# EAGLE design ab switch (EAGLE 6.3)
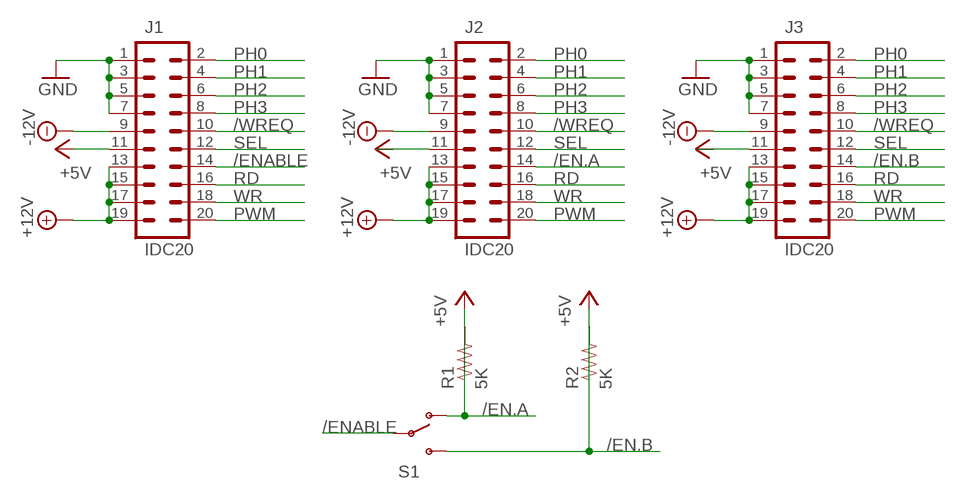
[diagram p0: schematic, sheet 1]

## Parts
J1  IDC20  [IDC20]
J2  IDC20  [IDC20]
J3  IDC20  [IDC20]
R1  5K  RESISTORPTH-1/4W  [AXIAL-0.4]
R2  5K  RESISTORPTH-1/4W  [AXIAL-0.4]
S1  SWITCH-SPDTPTH  [SWITCH-SPDT]

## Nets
+5V: J1.11 J2.11 J3.11 R1.P$1 R2.P$1
+12V: J1.13 J1.15 J1.17 J1.19 J2.13 J2.15 J2.17 J2.19 J3.13 J3.15 J3.17 J3.19
-12V: J1.9 J2.9 J3.9
/EN.A: J2.14 R1.P$2 S1.1(O)
/EN.B: J3.14 R2.P$2 S1.3(S)
/ENABLE: J1.14 S1.2(P)
/WREQ: J1.10 J2.10 J3.10
GND: J1.1 J1.3 J1.5 J1.7 J2.1 J2.3 J2.5 J2.7 J3.1 J3.3 J3.5 J3.7
PH0: J1.2 J2.2 J3.2
PH1: J1.4 J2.4 J3.4
PH2: J1.6 J2.6 J3.6
PH3: J1.8 J2.8 J3.8
PWM: J1.20 J2.20 J3.20
RD: J1.16 J2.16 J3.16
SEL: J1.12 J2.12 J3.12
WR: J1.18 J2.18 J3.18

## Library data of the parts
J1-J3 = big-mess-o-wires:IDC20
R1 R2 = SparkFun-Resistors:RESISTOR: Resistor
S1 = SparkFun-Electromechanical:SWITCH-SPDT: SPDT Switch Simple slide switch, Spark Fun Electronics SKU : COM-00102 DPDT SMT slide switch, AYZ0202, SWCH-08179

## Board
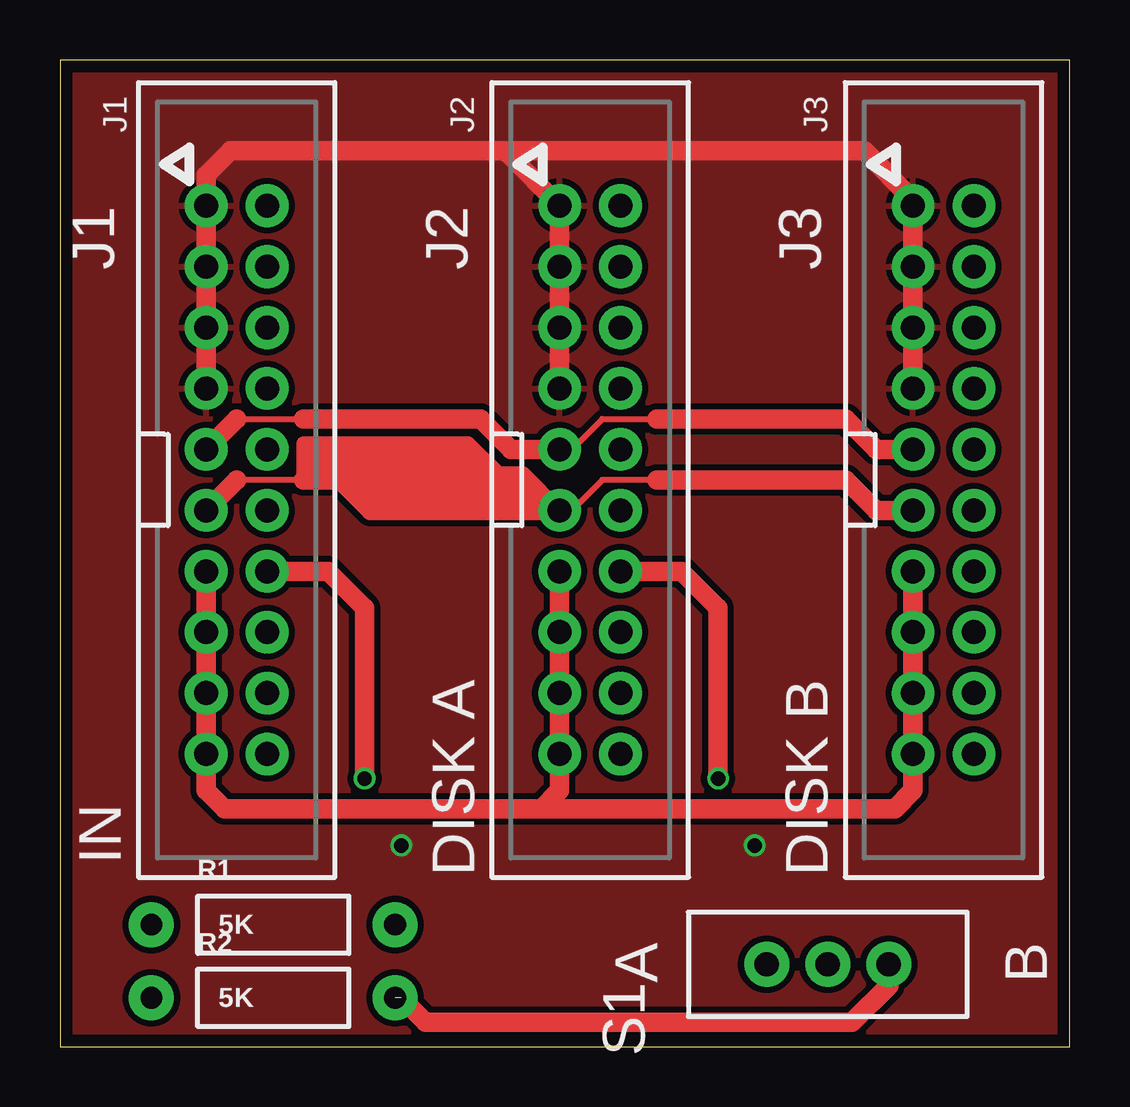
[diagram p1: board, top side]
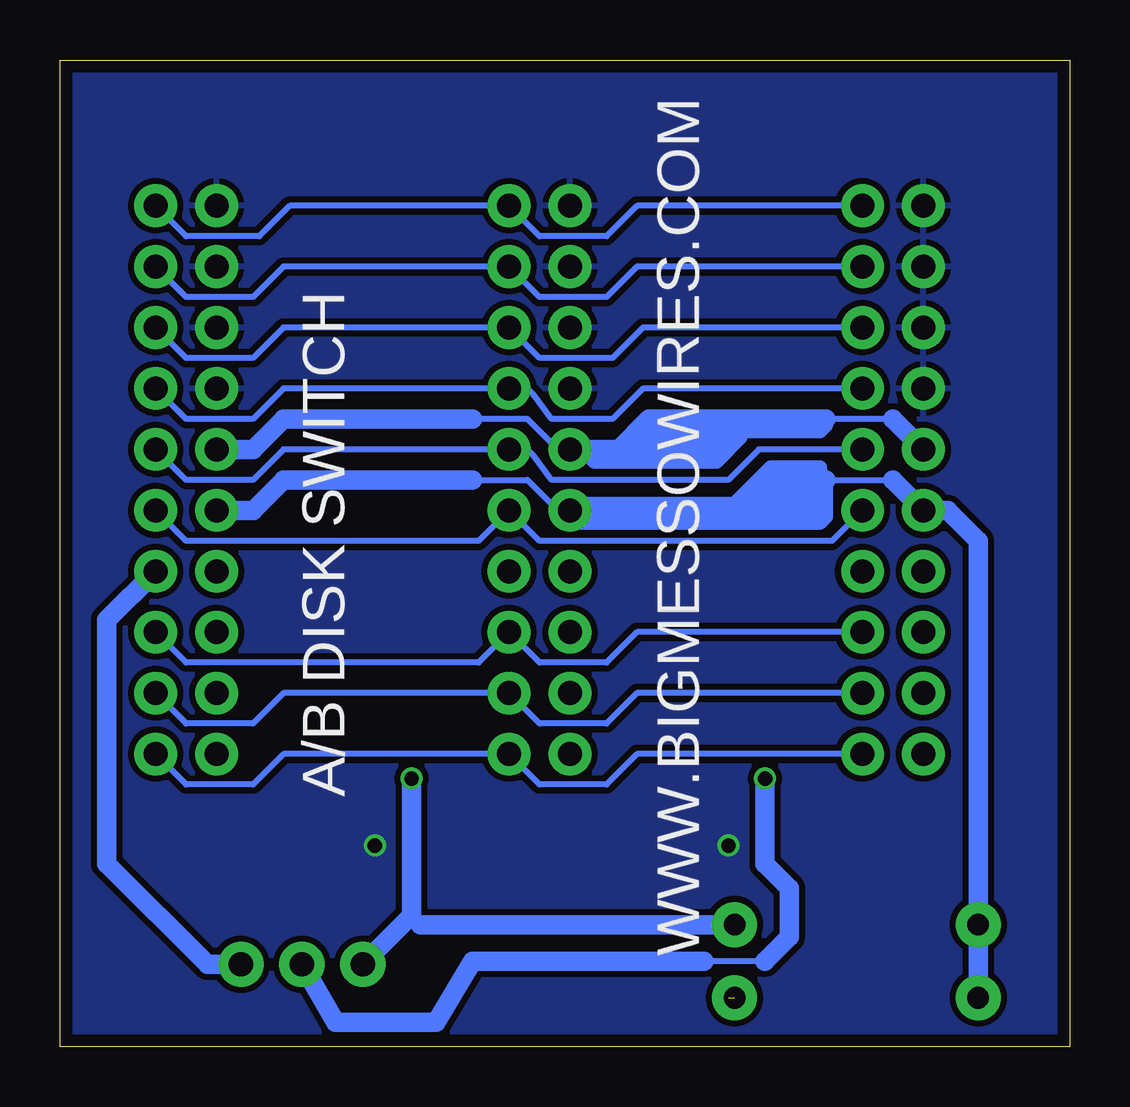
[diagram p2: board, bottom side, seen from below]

Size 42.09 x 41.13 mm. Coordinates in mm from the lower left corner, seen from the top.
Outline: 0,0 42.09,0 42.09,41.13 0,41.13 0,0
Copper layers (1*16): Top 0.035mm / dielectric 1.5mm / Bottom 0.035mm
Design rules "smart-prototyping": minimum track width 7mil, minimum drill 12mil, track to track 7mil, track to pad 7mil, pad to pad 7mil, via to via 7mil, smd to smd 0mil, copper to edge 20mil, drill to drill 10mil, minimum pad ring 10mil, minimum via ring 6mil, stop-mask expansion 2mil, vias tented up to drill 25mil, thermal gap 10mil

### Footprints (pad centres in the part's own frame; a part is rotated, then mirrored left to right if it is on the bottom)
IDC20 = drill 1 pad 1.778: 1 -11.43,-1.27; 2 -11.43,1.27; 3 -8.89,-1.27; 4 -8.89,1.27; 5 -6.35,-1.27; 6 -6.35,1.27; 7 -3.81,-1.27; 8 -3.81,1.27; 9 -1.27,-1.27; 10 -1.27,1.27; 11 1.27,-1.27; 12 1.27,1.27; 13 3.81,-1.27; 14 3.81,1.27; 15 6.35,-1.27; 16 6.35,1.27; 17 8.89,-1.27; 18 8.89,1.27; 19 11.43,-1.27; 20 11.43,1.27
AXIAL-0.4 = drill 0.9 pad 1.88: P$1 -5.08,0; P$2 5.08,0
SWITCH-SPDT = drill 1.016 pad 1.88: 1 0,2.54; 2 0,0; 3 0,-2.54

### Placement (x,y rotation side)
J1  7.37,23.62 270 top
J2  22.1,23.62 270 top
J3  36.83,23.62 270 top
R1  8.89,5.08 0 top
R2  8.89,2.03 0 top
S1  32,3.43 90 top

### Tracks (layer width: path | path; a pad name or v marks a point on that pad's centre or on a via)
+5V
  Top 0.254: 9.91,23.62 7.37,23.62 | 24.89,23.62 22.61,23.62 21.34,22.35
  Top 0.61: 10.16,23.62 10.16,25.15 17.02,25.15 18.29,23.88 19.3,23.88 J2.11 20.32,22.35 19.56,23.11
  Top 0.813: J1.11 7.37,23.62 | J2.11 12.95,22.35 11.68,23.62 10.16,23.62 | J3.11 34.04,22.35 32.77,23.62 24.89,23.62 | 19.56,23.11 12.95,23.11 11.68,24.38 10.67,24.38 10.67,24.64 16.76,24.64 17.53,23.88 17.78,23.88 18.03,23.62 | 18.03,23.62 18.8,23.62 | 18.03,23.62 17.27,23.62 17.02,23.88 12.45,23.88
  Bottom 0.254: J2.11 21.34,22.35 22.61,23.62 24.89,23.62 | 10.16,23.62 7.37,23.62
  Bottom 0.61: 10.16,23.62 10.16,22.1 10.41,21.84 20.32,21.84 J2.11 | J2.11 10.41,22.35 10.41,23.62 10.41,24.13 12.45,24.13 13.72,22.86 10.67,22.86 10.92,23.11 11.68,23.11 12.19,23.62 12.45,23.62 12.7,23.37 13.21,23.37 13.97,22.61 20.57,22.61 J2.11
  Bottom 0.813: 7.37,23.62 J1.11 5.08,22.35 3.81,21.08 R1.P$1 R2.P$1 | J2.11 12.95,22.35 11.68,23.62 10.41,23.62 10.16,23.62 | J3.11 34.04,22.35 32.77,23.62 24.89,23.62
+12V
  Top 0.813: J1.13 J1.15 J1.17 J1.19 6.1,10.67 6.86,9.91 20.07,9.91 | 20.07,9.91 20.83,10.67 J2.19 J2.17 J2.15 J2.13 | 20.07,9.91 34.8,9.91 35.56,10.67 J3.19 J3.17 J3.15 J3.13
-12V
  Top 0.254: 21.08,24.89 21.34,24.89 22.61,26.16 24.89,26.16 | 7.37,26.16 10.16,26.16
  Top 0.813: J3.9 34.04,24.89 32.77,26.16 24.89,26.16 | J1.9 7.37,26.16 | 21.08,24.89 18.8,24.89 17.53,26.16 10.16,26.16
  Bottom 0.254: J2.9 21.34,24.89 22.61,26.16 24.89,26.16 | 7.37,26.16 10.16,26.16
  Bottom 0.61: 10.16,26.16 10.16,25.91 10.41,25.65 13.72,25.65 | 13.97,25.65 13.72,25.65 | 13.72,25.65 13.72,25.4 14.73,24.38 19.81,24.38 20.07,24.64
  Bottom 0.813: J1.9 7.37,26.16 | 18.8,24.89 17.53,26.16 10.16,26.16 | 18.8,24.89 J2.9 | J3.9 34.04,24.89 32.77,26.16 24.89,26.16 | 18.8,24.89 14.99,24.89 14.22,25.65 17.27,25.65 17.53,25.4
/EN.A  (via drill 0.6)
  Top 0.813: J2.14 25.91,19.81 27.43,18.29 v27.43,11.18
  Bottom 0.254: 27.05,5.08 27.43,5.46
  Bottom 0.813: v27.43,11.18 27.43,5.46 S1.1 | R1.P$2 27.05,5.08
/EN.B  (1 unrouted)
  Top 0.813: 14.22,2.03 15.24,1.02 33.02,1.02 34.54,2.54 S1.3
  Bottom 0.813: S1.3 35.94,3.43 40.13,7.62 40.13,17.78 J3.14
/ENABLE  (via drill 0.6)
  Top 0.813: J1.14 11.18,19.81 12.7,18.29 v12.7,11.18
  Bottom 0.254: 12.7,3.56 15.24,3.56
  Bottom 0.813: v12.7,11.18 12.7,7.62 11.68,6.6 11.68,4.57 12.7,3.56 | S1.2 30.61,1.02 26.42,1.02 24.89,3.56 15.24,3.56
/WREQ
  Bottom 0.254: J1.10 12.95,24.89 14.22,23.62 21.59,23.62 22.35,24.64 22.61,24.89 J2.10 32.77,24.89 34.04,23.62 36.83,23.62 J3.10
GND  (via drill 0.6)
  Top 0.813: J1.7 J1.5 J1.3 J1.1 6.1,36.32 7.11,37.34 18.54,37.34 18.67,37.21 | 18.67,37.21 J2.1 J2.3 J2.5 J2.7 | 18.67,37.21 18.8,37.34 33.53,37.34 35.56,35.31 J3.1 J3.3 J3.5 J3.7
  other vias: 14.22,8.38 28.96,8.38
  pour Bottom (isolate 0.254): 0.51,0.51 41.66,0.51 41.66,40.64 0.51,40.64
  pour Top (isolate 0.254): 0.51,0.51 41.66,0.51 41.66,40.64 0.51,40.64
PH0
  Bottom 0.254: J1.2 18.03,35.05 19.3,33.78 22.1,33.78 J2.2 32.51,35.05 33.78,33.78 36.83,33.78 J3.2
PH1
  Bottom 0.254: J1.4 18.03,32.51 19.3,31.24 22.1,31.24 J2.4 32.77,32.51 34.04,31.24 36.83,31.24 J3.4
PH2
  Bottom 0.254: J1.6 17.78,29.97 19.05,28.7 22.1,28.7 J2.6 32.77,29.97 34.04,28.7 36.83,28.7 J3.6
PH3
  Bottom 0.254: J1.8 17.78,27.43 19.05,26.16 21.59,26.16 22.35,27.18 22.61,27.43 J2.8 32.77,27.43 34.04,26.16 36.83,26.16 J3.8
PWM
  Bottom 0.254: J1.20 18.03,12.19 19.3,10.92 22.1,10.92 J2.20 32.77,12.19 34.04,10.92 36.83,10.92 J3.20
RD
  Bottom 0.254: J1.16 18.03,17.27 19.3,16 22.1,16 J2.16 24.64,16 36.83,16 J3.16
SEL
  Bottom 0.254: J1.12 9.91,21.08 22.1,21.08 J2.12 24.64,21.08 36.83,21.08 J3.12
WR
  Bottom 0.254: J1.18 18.03,14.73 19.3,13.46 22.1,13.46 J2.18 32.77,14.73 34.04,13.46 36.83,13.46 J3.18

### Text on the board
tPlace: J1 | J2 | J3 | IN | DISK A | DISK B | A | B
bPlace: WWW.BIGMESSOWIRES.COM | A/B DISK SWITCH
